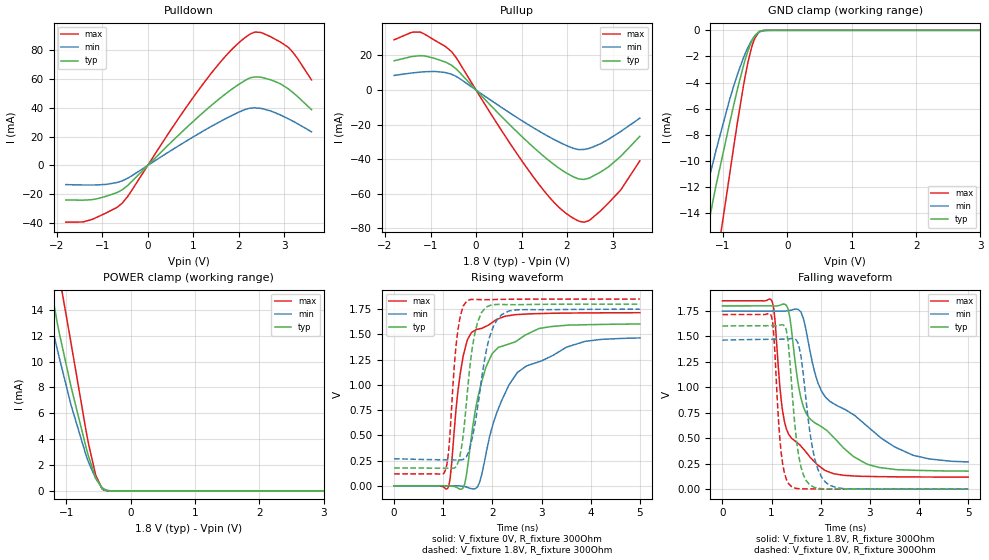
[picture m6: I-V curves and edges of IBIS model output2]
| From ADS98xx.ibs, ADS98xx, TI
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|   output2 Model
[Model]   output2
Model_type   Output
Polarity   Non-Inverting
Vmeas = 0.9
Vref = 0
Cref = 2pF
Rref = 100000
|   typ   min   max
C_comp   0.608pF   0.518pF   0.645pF
[Voltage Range]   1.8   1.75   1.85
[Temperature Range]   27   125   -40
[Pullup Reference]   1.8   1.75   1.85
[Pulldown Reference]   0   0   0
[Power Clamp Reference]   1.8   1.75   1.85
[GND Clamp Reference]   0   0   0
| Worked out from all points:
|   slope of the pulldown table from 0 to 0.27 V, typ, clamps not added: 31.7 ohm
|   slope of the pullup table from 0 to 0.27 V, typ, clamps not added: 36.1 ohm
|   GND clamp passes 1 mA (typ) near -0.57 V on its own axis
|   POWER clamp passes 1 mA (typ) near -0.54 V on its own axis
|   falling waveform, V_fixture 1.8V, R_fixture 300Ohm: 20-80 % time 852ps typ, 1.33ns min, 406ps max; typ from 1.8 V to 0.177 V
|   rising waveform, V_fixture 0V, R_fixture 300Ohm: 20-80 % time 439ps typ, 790ps min, 260ps max; typ from 0 V to 1.6 V
|   rising waveform, V_fixture 1.8V, R_fixture 300Ohm: 20-80 % time 224ps typ, 305ps min, 160ps max; typ from 0.177 V to 1.8 V
|   falling waveform, V_fixture 0V, R_fixture 300Ohm: 20-80 % time 186ps typ, 248ps min, 136ps max; typ from 1.6 V to 0 V
[Pulldown]
|   Voltage   I(typ)   I(min)   I(max)
-1.8V     -23.88mA   -13.25mA   -39.29mA
-1.228V   -23.69mA   -13.54mA   -37.45mA
-558mV    -16.78mA   -10.62mA   -26.01mA
689.4mV   21.35mA    13.81mA    33.11mA
1.251V    37.57mA    24.4mA     57.89mA
1.823V    52.22mA    34.18mA    79.52mA
2.266V    60.8mA     39.73mA    91.25mA
2.52V     60.89mA    39.34mA    91.74mA
2.92V     56.53mA    34.94mA    85.4mA
3.092V    53mA       32.31mA    81.79mA
3.292V    47.79mA    28.96mA    74.16mA
3.6V      38.65mA    23.32mA    59.25mA
[GND Clamp]
|   Voltage   I(typ)   I(min)   I(max)
-1.8V     -32.32mA   -23.42mA   -46.74mA
-1.422V   -20.52mA   -15.48mA   -29.34mA
-1.363V   -18.74mA   -14.26mA   -26.85mA
-1.228V   -14.85mA   -11.53mA   -21.89mA
-1.109V   -11.85mA   -9.169mA   -17.96mA
-909mV    -7.348mA   -5.491mA   -11.39mA
-682.2mV  -2.692mA   -2.095mA   -4.219mA
-612mV    -1.557mA   -1.298mA   -2.425mA
-558mV    -868.8uA   -798uA     -1.33mA
-504mV    -388.2uA   -421.2uA   -573.4uA
-444.6mV  -111.2uA   -164.4uA   -149.2uA
3.6V      0A         0A         0A
[Pullup]
|   Voltage   I(typ)   I(min)   I(max)
-1.8V     16.93mA    8.447mA    29.04mA
-1.433V   19.23mA    9.788mA    33.16mA
-1.228V   19.84mA    10.36mA    33.49mA
-541.8mV  14.38mA    9.133mA    22.27mA
613.8mV   -16.74mA   -11mA      -25.54mA
1.278V    -33.47mA   -22.08mA   -50.86mA
1.807V    -44.88mA   -29.83mA   -67.41mA
2.207V    -50.92mA   -34.17mA   -75.1mA
2.455V    -51.17mA   -33.95mA   -75.78mA
2.731V    -47.51mA   -31.13mA   -70.02mA
3.19V     -38.07mA   -23.8mA    -57.41mA
3.6V      -26.78mA   -16.27mA   -40.94mA
[POWER Clamp]
|   Voltage   I(typ)   I(min)   I(max)
-1.8V     35.23mA    25.8mA     50.55mA
-1.384V   20.4mA     16.22mA    27.35mA
-1.319V   18.26mA    14.78mA    24.19mA
-1.217V   15.08mA    12.54mA    19.93mA
-1.12V    12.41mA    10.48mA    16.87mA
-930.6mV  8.119mA    6.697mA    11.51mA
-671.4mV  2.952mA    2.434mA    4.039mA
-541.8mV  973.2uA    940.7uA    1.196mA
-444.6mV  178.5uA    258.9uA    159.2uA
-423mV    104.7uA    174.5uA    84.17uA
-217.8mV  96.71nA    978.9nA    54.24nA
3.6V      0A         0A         0A
[Ramp]
R_load = 300
|   typ   min   max
dV/dt_r   0.961671/4.38721e-10   0.878602/7.89517e-10   1.02882/2.59802e-10
dV/dt_f   0.973502/8.52081e-10   0.88898/1.33391e-09   1.039/4.05624e-10
[Falling Waveform]
V_fixture = 1.8V
V_fixture_min = 1.75V
V_fixture_max = 1.85V
R_fixture = 300Ohm
C_fixture = 0F
|   Time   V(typ)   V(min)   V(max)
0s        1.8V       1.749V     1.85V
998.9ps   1.8V       1.75V      1.854V
1.068ns   1.799V     1.75V      1.663V
1.195ns   1.811V     1.749V     873.6mV
1.3ns     1.805V     1.75V      593.2mV
1.644ns   813.1mV    1.679V     396.6mV
2.081ns   591mV      914.5mV    185.4mV
2.945ns   244.7mV    618.5mV    125.4mV
3.879ns   186.1mV    333mV      120.2mV
5ns       177.2mV    267.6mV    118.2mV
[Rising Waveform]
V_fixture = 0V
V_fixture_min = 0V
V_fixture_max = 0V
R_fixture = 300Ohm
C_fixture = 0F
|   Time   V(typ)   V(min)   V(max)
0s        142.5uV    333.7uV    55.88uV
1.087ns   190.2uV    184.6uV    -27.25mV
1.137ns   -1.024mV   274.1uV    62.82mV
1.4ns     -24.15mV   -5.136mV   1.27V
1.573ns   487.4mV    -28.84mV   1.519V
1.732ns   933.5mV    26.25mV    1.555V
1.994ns   1.309V     578.3mV    1.617V
2.508ns   1.44V      1.122V     1.697V
3.879ns   1.595V     1.43V      1.713V
5ns       1.603V     1.465V     1.715V
[Rising Waveform]
V_fixture = 1.8V
V_fixture_min = 1.75V
V_fixture_max = 1.85V
R_fixture = 300Ohm
C_fixture = 0F
|   Time   V(typ)   V(min)   V(max)
0s        177.2mV    266.7mV    118.3mV
1.044ns   174.5mV    256.8mV    156.3mV
1.111ns   174mV      256.4mV    354.1mV
1.224ns   176.7mV    255.7mV    1.186V
1.3ns     229.8mV    255.1mV    1.55V
1.489ns   916.9mV    305.7mV    1.836V
1.701ns   1.624V     786.2mV    1.845V
1.944ns   1.784V     1.477V     1.844V
2.187ns   1.796V     1.695V     1.847V
5ns       1.8V       1.749V     1.85V
[Falling Waveform]
|Gnd
V_fixture = 0V
V_fixture_min = 0V
V_fixture_max = 0V
R_fixture = 300Ohm
C_fixture = 0F
|   Time   V(typ)   V(min)   V(max)
0s        1.603V     1.464V     1.715V
998.9ps   1.605V     1.472V     1.695V
1.195ns   1.613V     1.473V     355mV
1.299ns   1.563V     1.474V     98.92mV
1.407ns   1.029V     1.479V     24.36mV
1.512ns   456.4mV    1.458V     7.195mV
1.644ns   144mV      1.13V      3.238mV
1.836ns   26.56mV    390.7mV    2.509mV
2.096ns   2.922mV    68.74mV    1.148mV
5ns       142.4uV    324.4uV    55.82uV
